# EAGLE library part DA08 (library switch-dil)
DIL/CODE SWITCH
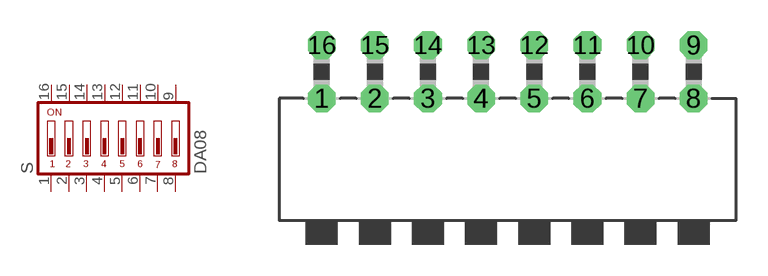
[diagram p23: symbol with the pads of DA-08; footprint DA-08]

Designator prefix S

## DA08 (MPN: MCDA08; OC_FARNELL: 9471561; OC_NEWARK: 26M1092)  [DA-08]
1  1  pas
2  2  pas
3  3  pas
4  4  pas
5  5  pas
6  6  pas
7  7  pas
8  8  pas
9  9  pas
10  10  pas
11  11  pas
12  12  pas
13  13  pas
14  14  pas
15  15  pas
16  16  pas

## Footprint DA-08 (pad centres in mm)
DIL/CODE SWITCH Mors distributor Buerklin, 17G592
drill 0.813 octagon: 1 -8.89,-1.27; 2 -6.35,-1.27; 3 -3.81,-1.27; 4 -1.27,-1.27; 5 1.27,-1.27; 6 3.81,-1.27; 7 6.35,-1.27; 8 8.89,-1.27; 9 8.89,1.27; 10 6.35,1.27; 11 3.81,1.27; 12 1.27,1.27; 13 -1.27,1.27; 14 -3.81,1.27; 15 -6.35,1.27; 16 -8.89,1.27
